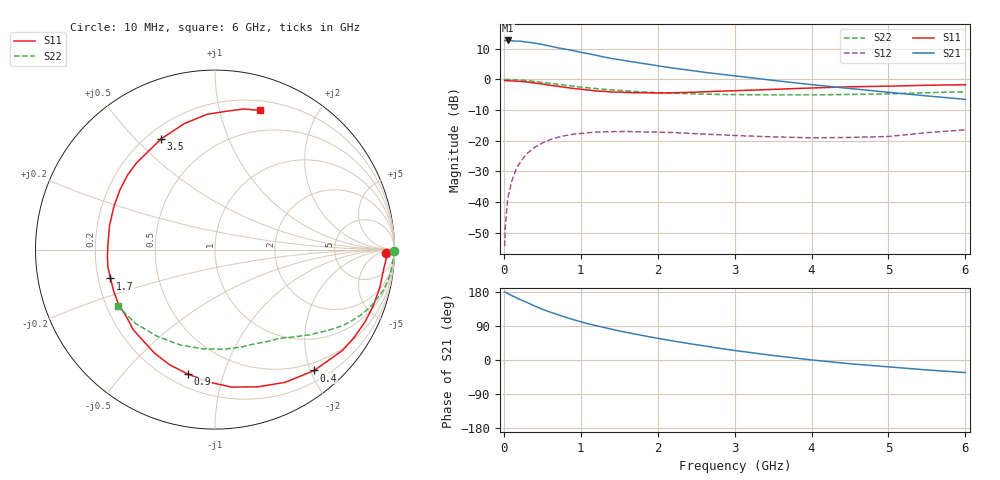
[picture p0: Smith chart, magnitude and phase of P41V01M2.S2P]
! SIEMENS Small Signal Semiconductors
! BFP182
! Si NPN RF Bipolar Junction Transistor in SOT143
! VCE = 1 V  IC = 1.2 mA
! Common Emitter S-Parameters:  March  1996
# GHz  S  MA  R  50
!  f  S11  S21  S12  S22
! GHz  MAG  ANG  MAG  ANG  MAG  ANG  MAG  ANG
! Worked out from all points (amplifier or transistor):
!   36 points, 10 MHz to 6 GHz, reference 50 ohm
!   highest |S21| = 12.7 dB at 50 MHz (marker M1)
!   |S21| within 3 dB of that: start of sweep to 832.8 MHz
!   unconditionally stable (mu >= 1): 2.449 GHz to end of sweep
!   at 250 MHz: K = 0.10, MSG = 19.0 dB, |S12| = -25.8 dB
!   at 1.4 GHz: K = 0.59, MSG = 11.9 dB, |S12| = -17.1 dB
!   at 6 GHz: K = 1.18, MAG = 2.4 dB, |S12| = -16.5 dB
!   S11 on the Smith chart (normalised r, x): 10 MHz: 34, -16; 400 MHz: 0.37, -2.06; 900 MHz: 0.27, -0.77; 1.7 GHz: 0.25, -0.13; 3.5 GHz: 0.26, +0.59; 6 GHz: 0.29, +1.33
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0.01  0.9534 -1.3  4.267 179.4  0.0019 90.1  0.9973 -0.5
0.02  0.9557 -2.8  4.267 178.7  0.0042 89.4  0.9915 -1.0
0.05  0.9462 -6.6  4.302 175.2  0.0113 87.5  0.9954 -2.6
0.1  0.9425 -12.9  4.247 170.4  0.0212 80.4  0.9898 -5.3
0.15  0.9356 -19.8  4.193 165.5  0.0321 77.4  0.9858 -8.0
0.2  0.9275 -26.0  4.208 160.6  0.0421 74.4  0.977 -10.5
0.4  0.8713 -50.6  3.901 142.4  0.0776 59.6  0.9254 -19.8
0.5  0.8368 -62.1  3.695 134.0  0.0915 52.6  0.893 -23.9
0.6  0.8005 -72.8  3.488 126.6  0.1034 46.8  0.8603 -27.4
0.8  0.7388 -92.7  3.099 112.9  0.1208 36.7  0.8004 -33.2
0.9  0.71 -102.2  2.939 106.8  0.1271 32.4  0.7729 -35.6
1.1  0.6683 -120.2  2.619 95.4  0.1348 24.5  0.7254 -40.1
1.4  0.6193 -142.7  2.187 81.3  0.14 15.2  0.6737 -45.8
1.7  0.6043 -164.6  1.903 68.7  0.1402 8.8  0.6347 -50.5
1.9  0.6006 -176.5  1.743 61.0  0.1383 5.5  0.6147 -53.7
2.2  0.6026 167.2  1.523 50.1  0.1351 1.2  0.5959 -58.5
2.8  0.6401 139.6  1.217 30.9  0.1246 -3.2  0.5658 -69.4
3.5  0.6854 116.1  0.961 11.9  0.115 -3.7  0.5578 -84.6
4  0.7223 103.8  0.82 0.2  0.1113 -0.5  0.5574 -97.1
4.5  0.7553 93.3  0.708 -9.9  0.1126 2.7  0.5659 -110.3
5.5  0.7998 78.4  0.536 -26.3  0.1349 9.6  0.6045 -137.0
6  0.815 72.1  0.471 -33.2  0.1499 8.4  0.6256 -149.9
